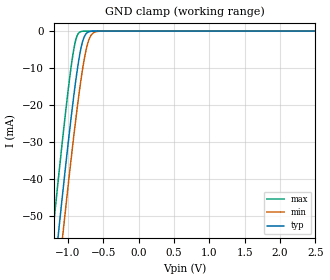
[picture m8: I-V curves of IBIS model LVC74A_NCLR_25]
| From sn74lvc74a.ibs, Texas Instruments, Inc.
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[Model]   LVC74A_NCLR_25
Model_type  Input
Vinl=0.7
Vinh=1.7
| variable   typ   min   max
C_comp   4.83pF   3.85pF   5.99pF
[Temperature Range]   40   100   -40
| Ambient temperature   25   85   -40
[Voltage range]   2.5   2.3   2.7
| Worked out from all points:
|   GND clamp passes 1 mA (typ) near -0.75 V on its own axis
[GND Clamp]
| LVC74A_NCLR_25
|   Voltage   I(typ)   I(min)   I(max)
-5.5V     -915.9mA   -925.7mA   -903.9mA
-1.215V   -69.33mA   -80.91mA   -54.47mA
-1.14V    -55.53mA   -67.11mA   -40.64mA
-1.075V   -43.82mA   -55.36mA   -29.01mA
-1.06V    -41.16mA   -52.69mA   -26.4mA
-960mV    -24.12mA   -35.32mA   -10.31mA
-885mV    -12.72mA   -23.13mA   -2.077mA
-830mV    -5.985mA   -15.02mA   -239.8uA
-780mV    -2.057mA   -8.704mA   -23.97uA
-720mV    -339uA     -3.291mA   -1.43uA
-650mV    -30.77uA   -620.5uA   -53.02nA
2.5V      4.714pA    8.54pA     4.389pA
